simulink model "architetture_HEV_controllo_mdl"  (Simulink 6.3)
settings: Solver=ode45  StartTime=0.0  StopTime=8  RelTol=1e-3
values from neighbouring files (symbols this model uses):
  b_c = kb*J_c    (= 4.94590955184)    [architetture_epicicloidale.m]    (also in architetture_epicicloidale_cont.m; architetture_epicicloidale_HEV.m = 92.8974810391; architetture_epicicloidale_prova.m; architetture_HEV_controllo.m = 9.28974810391)
  b_p = kb*J_p    (= 8.12277148259)    [architetture_epicicloidale_HEV.m]    (also in architetture_HEV_controllo.m = 0.812277148259; architetture_HEV_startstop.m = 0.0731049433433; Confronto_CVT_EMR.m = 0; epicicloidale_confronto_statico_elastico.m)
  b_r = kb*J_r    (= 218.026030555)    [architetture_epicicloidale.m]    (also in architetture_epicicloidale_cont.m; architetture_epicicloidale_HEV.m; architetture_epicicloidale_prova.m; architetture_HEV_controllo.m = 21.8026030555)
  b_s = kb*J_s    (= 8.12277148259)    [architetture_epicicloidale.m]    (also in architetture_epicicloidale_cont.m; architetture_epicicloidale_HEV.m = 4.94590955184; architetture_epicicloidale_prova.m; architetture_HEV_controllo.m = 0.494590955184)
  bm = 0.8*N*metri*secondo/rad    (= 0.8)    [architetture_epicicloidale.m]    (also in architetture_epicicloidale_cont.m; architetture_epicicloidale_HEV.m; architetture_epicicloidale_prova.m; architetture_HEV_controllo.m)
  d_cr = d0    (= 10)    [architetture_epicicloidale_HEV.m]    (also in architetture_HEV_controllo.m = 1000; architetture_HEV_startstop.m = 90; epicicloidale_confronto_statico_elastico.m; epicicloidale_statico.m)
  d_sc = d0    (= 10)    [architetture_epicicloidale_HEV.m]    (also in architetture_HEV_controllo.m = 1000; architetture_HEV_startstop.m = 90; epicicloidale_confronto_statico_elastico.m; epicicloidale_statico.m)
  I_m = eye(m-1)    [architetture_epicicloidale.m]    (also in architetture_epicicloidale_cont.m; architetture_epicicloidale_HEV.m; architetture_epicicloidale_prova.m; architetture_HEV_controllo.m)
  Iw0 = 0*wI0    [architetture_epicicloidale.m]    (also in architetture_epicicloidale_cont.m = wI0; architetture_epicicloidale_HEV.m; architetture_epicicloidale_prova.m; architetture_HEV_controllo.m)
  J_c = 1.3*0.5*pi*rho_acc*hc*r_c^4    (= 0.0494590955184)    [architetture_epicicloidale.m]    (also in architetture_epicicloidale_cont.m; architetture_epicicloidale_HEV.m = 0.928974810391; architetture_epicicloidale_prova.m; architetture_HEV_controllo.m = 0.928974810391)
  J_p = Nr_sat*0.5*pi*rho_acc*(hs*r_p^4 + hc*r_p^4)    (= 0.0812277148259)    [architetture_epicicloidale_HEV.m]    (also in architetture_HEV_controllo.m; architetture_HEV_startstop.m; Confronto_CVT_EMR.m = 0; epicicloidale_confronto_statico_elastico.m)
  J_r = 0.5*pi*rho_acc*(hr*r_ri^4 + h_ring*(r_re^4-r_ri^4))    (= 2.18026030555)    [architetture_epicicloidale.m]    (also in architetture_epicicloidale_cont.m; architetture_epicicloidale_HEV.m; architetture_epicicloidale_prova.m; architetture_HEV_controllo.m)
  J_s = Nr_sat*0.5*pi*rho_acc*(hs*r_s^4 + hc*r_s^4)    (= 0.0812277148259)    [architetture_epicicloidale.m]    (also in architetture_epicicloidale_cont.m; architetture_epicicloidale_HEV.m = 0.0494590955184; architetture_epicicloidale_prova.m; architetture_HEV_controllo.m = 0.0494590955184)
  Jm = 1.6*kg*metri^2    (= 1.6)    [architetture_epicicloidale.m]    (also in architetture_epicicloidale_cont.m; architetture_epicicloidale_HEV.m = 1.64945909552; architetture_epicicloidale_prova.m; architetture_HEV_controllo.m = 0.529459095518)
  Jr = Jr([1:m-1],[1:m-1])    [architetture_epicicloidale.m]    (also in architetture_epicicloidale_cont.m; architetture_epicicloidale_HEV.m; architetture_epicicloidale_prova.m; architetture_HEV_controllo.m)
  K_cr = K0    (= 10000)    [architetture_epicicloidale_HEV.m]    (also in architetture_HEV_controllo.m = 100000; architetture_HEV_startstop.m = 10000000; epicicloidale_confronto_statico_elastico.m; epicicloidale_statico.m)
  K_sc = K0    (= 10000)    [architetture_epicicloidale_HEV.m]    (also in architetture_HEV_controllo.m = 100000; architetture_HEV_startstop.m = 10000000; epicicloidale_confronto_statico_elastico.m; epicicloidale_statico.m)
  Kf = diag(diag(MLb)'./fliplr(tau_m(1:m-1)))    [architetture_epicicloidale_cont.m]    (also in architetture_epicicloidale_HEV.m; architetture_epicicloidale_prova.m; architetture_HEV_controllo.m; architetture_HEV_startstop.m)
  Kr = Kr([1:m-1])    [architetture_epicicloidale.m]    (also in architetture_epicicloidale_cont.m; architetture_epicicloidale_HEV.m; architetture_epicicloidale_prova.m; architetture_HEV_controllo.m)
  Li = 0.1*Henry    (= 0.1)    [architetture_epicicloidale.m]    (also in architetture_epicicloidale_cont.m; architetture_epicicloidale_HEV.m; architetture_epicicloidale_prova.m; architetture_HEV_controllo.m)
  m = 5    [architetture_epicicloidale.m]    (also in architetture_epicicloidale_cont.m; architetture_epicicloidale_HEV.m; architetture_epicicloidale_prova.m; architetture_HEV_controllo.m)
  Mi = 0.08*Henry    (= 0.08)    [architetture_epicicloidale.m]    (also in architetture_epicicloidale_cont.m; architetture_epicicloidale_HEV.m; architetture_epicicloidale_prova.m; architetture_HEV_controllo.m)
  MKr = MKr([1:m-1],[1:m-1])    [architetture_epicicloidale.m]    (also in architetture_epicicloidale_cont.m; architetture_epicicloidale_HEV.m; architetture_epicicloidale_prova.m; architetture_HEV_controllo.m)
  MLb = MLb([1:m-1],[1:m-1])    [architetture_epicicloidale.m]    (also in architetture_epicicloidale_cont.m; architetture_epicicloidale_HEV.m; architetture_epicicloidale_prova.m; architetture_HEV_controllo.m)
  MR = MR([1:m-1],[1:m-1])    [architetture_epicicloidale.m]    (also in architetture_epicicloidale_cont.m; architetture_epicicloidale_HEV.m; architetture_epicicloidale_prova.m; architetture_HEV_controllo.m)
  Nar = 200    [architetture_epicicloidale.m]    (also in architetture_epicicloidale_cont.m; architetture_epicicloidale_HEV.m; architetture_epicicloidale_prova.m; architetture_HEV_controllo.m)
  Nc = 30    [architetture_epicicloidale.m]    (also in architetture_epicicloidale_cont.m; architetture_epicicloidale_HEV.m; architetture_epicicloidale_prova.m; architetture_HEV_controllo.m)
  Nr_sat = 4    [architetture_epicicloidale.m]    (also in architetture_epicicloidale_cont.m; architetture_epicicloidale_HEV.m; architetture_epicicloidale_prova.m; architetture_HEV_controllo.m)
  p = 1    [architetture_epicicloidale.m]    (also in architetture_epicicloidale_cont.m; architetture_epicicloidale_HEV.m; architetture_epicicloidale_prova.m; architetture_HEV_controllo.m)
  Phir = 0.02*Weber    (= 0.02)    [architetture_epicicloidale.m]    (also in architetture_epicicloidale_cont.m; architetture_epicicloidale_HEV.m; architetture_epicicloidale_prova.m; architetture_HEV_controllo.m)
  r_p = xds*Np/(2*pi)    (= 0.0732112738223)    [architetture_epicicloidale_HEV.m]    (also in architetture_HEV_controllo.m; architetture_HEV_startstop.m; Confronto_CVT_EMR.m = 0.025; epicicloidale_confronto_statico_elastico.m)
  r_r = xds*Nr/(2*pi)    (= 0.248281711223)    [architetture_epicicloidale_HEV.m]    (also in architetture_HEV_controllo.m; architetture_HEV_startstop.m; Confronto_CVT_EMR.m = 0.1; epicicloidale_confronto_statico_elastico.m)
  r_s = xds*Ns/(2*pi)    (= 0.0732112738223)    [architetture_epicicloidale.m]    (also in architetture_epicicloidale_cont.m; architetture_epicicloidale_HEV.m = 0.101859163579; architetture_epicicloidale_prova.m; architetture_HEV_controllo.m = 0.101859163579)
  Ri = 3*Ohm    (= 3)    [architetture_epicicloidale.m]    (also in architetture_epicicloidale_cont.m; architetture_epicicloidale_HEV.m; architetture_epicicloidale_prova.m; architetture_HEV_controllo.m = 0.1)
  Star = Si    [architetture_epicicloidale.m]    (also in architetture_epicicloidale_cont.m; architetture_epicicloidale_HEV.m; architetture_epicicloidale_prova.m; architetture_HEV_controllo.m)
  Tau_stop = 10000000    [architetture_HEV_controllo.m]
  Tc = 0.05*ms    (= 5e-05)    [architetture_epicicloidale.m]    (also in architetture_epicicloidale_cont.m; architetture_epicicloidale_HEV.m; architetture_epicicloidale_prova.m; architetture_HEV_controllo.m)
  Tc_0 = 0*N*metri    (= 0)    [architetture_epicicloidale_HEV.m]    (also in architetture_HEV_controllo.m; architetture_HEV_startstop.m; epicicloidale_confronto_statico_elastico.m; epicicloidale_statico.m)
  Thm0 = 0    [architetture_epicicloidale.m]    (also in architetture_epicicloidale_cont.m; architetture_epicicloidale_HEV.m; architetture_epicicloidale_prova.m; architetture_HEV_controllo.m)
  Tr_0 = 0*N*metri    (= 0)    [architetture_epicicloidale_HEV.m]    (also in architetture_HEV_controllo.m; architetture_HEV_startstop.m; epicicloidale_confronto_statico_elastico.m; epicicloidale_statico.m)
  Ts = Tfin/2000    (= 0.00025)    [architetture_epicicloidale.m]    (also in architetture_epicicloidale_cont.m = 0.001; architetture_epicicloidale_HEV.m = 0.0025; architetture_epicicloidale_prova.m = 0.001; architetture_HEV_controllo.m = 0.004)
  Ts_0 = 0*N*metri    (= 0)    [architetture_epicicloidale_HEV.m]    (also in architetture_HEV_controllo.m; architetture_HEV_startstop.m; epicicloidale_confronto_statico_elastico.m; epicicloidale_statico.m)
  tTb = tTb(:,[1:m-1])    [architetture_epicicloidale.m]    (also in architetture_epicicloidale_cont.m; architetture_epicicloidale_HEV.m; architetture_epicicloidale_prova.m; architetture_HEV_controllo.m)
  W_c = 100*rpm    (= 10.471975512)    [architetture_epicicloidale_HEV.m]    (also in architetture_HEV_controllo.m = 104.71975512; architetture_HEV_startstop.m = 0; PMSM_controllo_w.m; architetture_HEV_startstop_1.m = 0)
  Wm0 = 0*Wr_d    (= 0)    [architetture_epicicloidale.m]    (also in architetture_epicicloidale_cont.m = 62.5; architetture_epicicloidale_HEV.m; architetture_epicicloidale_prova.m; architetture_HEV_controllo.m)
undefined symbols (not defined in the file or in its folder): a_0, a_1, B_Pneumatico, DFKc_max, eps_sk, K_Pneumatico, Lambda_mu, Mass_Matrix, Massa_Corpo_Auto, Mu_lambda, Raggio_Ruota_Ant, Raggio_Ruota_Pos, T_omega, tau_a0
libraries: simulink x11, dspmtrx3 x4, Tire_Soil x2, planetary_gear_blocks x1, POG_Sincronous_Motors x1, dspstat3 x1

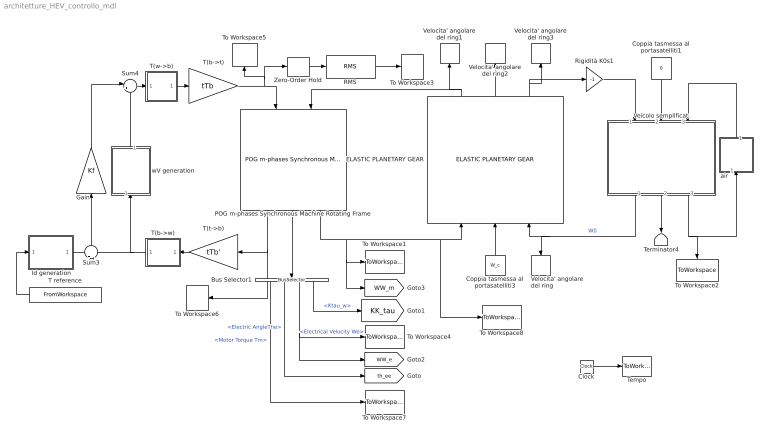
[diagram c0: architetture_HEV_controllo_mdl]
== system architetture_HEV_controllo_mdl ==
  " Id generation" : Subsystem
  Bus Selector1 : BusSelector  Orientation=down  OutputSignals=Motor Torque Tm,Electric AngleThe,Electrical Velocity We,Ktau_w
  Clock : Clock
  Coppia tasmessa al portasatelliti1 : Constant  Orientation=down  Value=0
  Coppia tasmessa al portasatelliti3 : Constant  Orientation=up  Value=W_c
  ELASTIC PLANETARY GEAR : planetary_gear_blocks/ELASTIC PLANETARY GEAR  Orientation=up  Par_solare=[J_s, b_s, r_s]  Par_satelliti=[J_p, J_c, b_p, b_c, r_p, Nr_sat]  Par_ring=[J_r, b_r, r_r]  Solare_Satelliti=[K_sc, d_sc]  Satelliti_Ring=[K_cr, d_cr]  Cond_in=[Ts_0, Tc_0, Tr_0]
  Gain : Gain  Orientation=up  Gain=Kf  Multiplication=Matrix(K*u) (u vector)
  POG m-phases Synchronous Machine Rotating Frame : POG_Sincronous_Motors/POG m-phases Synchronous Machine Rotating Frame  Orientation=down  Motor_Par=[m p]  Phase_Par=[Nc Star]  Electric_Par=[Ri Li Mi]  Mech_Par=[Jm bm]  Plux_Par=[Phir Nar]  Iniz_Cond=[Wm0; Thm0; Iw0]  TipoFlux=User defined  Tipo=Tipo  alfa=al  degree=6  TipoF=Tipo
  RMS : dspstat3/RMS  run=on  reset_popup=None
  Rigidità K0s1 : Gain  Gain=-1
  Sum3 : Sum  Orientation=up  Inputs=+|-
  Sum4 : Sum  Inputs=|++
  T reference : FromWorkspace  Orientation=left  VariableName=[T_in T_des]  SampleTime=0
  T(b->t) : Gain  Gain=tTb  Multiplication=Matrix(K*u) (u vector)
  T(b->w) : Subsystem  Orientation=left  AncestorBlock=|
      | POG_Electric_Bloks/POG m-phases
      | Synchronous Machine
      | Rotating Frame/T(b->w)
  T(t->b) : Gain  Orientation=left  Gain=tTb'  Multiplication=Matrix(K*u) (u vector)
  T(w->b) : Subsystem  AncestorBlock=|
      | POG_Electric_Bloks/POG m-phases
      | Synchronous Machine
      | Rotating Frame/T(w->b)
  Tempo : ToWorkspace  VariableName=t  SampleTime=Tc  SaveFormat=Array
  Terminator4 : Terminator
  To Workspace1 : ToWorkspace  VariableName=Wm  SampleTime=Tc  SaveFormat=Array
  To Workspace2 : ToWorkspace  VariableName=Vvehicle  SampleTime=Tc  SaveFormat=Array
  To Workspace3 : ToWorkspace  VariableName=Vt1  SampleTime=Tc  SaveFormat=Array
  To Workspace4 : ToWorkspace  VariableName=We  SampleTime=Tc  SaveFormat=Array
  To Workspace5 : ToWorkspace  VariableName=Vt  SampleTime=Tc  SaveFormat=Array
  To Workspace6 : ToWorkspace  VariableName=It  SampleTime=Tc  SaveFormat=Array
  To Workspace7 : ToWorkspace  VariableName=Tm  SampleTime=Tc  SaveFormat=Array
  To Workspace8 : ToWorkspace  VariableName=Ws  SampleTime=Tc  SaveFormat=Array
  Veicolo semplificat : Subsystem  Orientation=down
  Velocita' angolare del ring : ToWorkspace  VariableName=W_r  SampleTime=Tc  SaveFormat=Array
  Velocita' angolare del ring1 : ToWorkspace  VariableName=Tau_s  SampleTime=Tc  SaveFormat=Array
  Velocita' angolare del ring2 : ToWorkspace  VariableName=Tau_c  SampleTime=Tc  SaveFormat=Array
  Velocita' angolare del ring3 : ToWorkspace  VariableName=Tau_r  SampleTime=Tc  SaveFormat=Array
  Zero-Order Hold : ZeroOrderHold  SampleTime=Ts
  air : Subsystem  Orientation=up
  wV generation : Subsystem  Orientation=up
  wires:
  Clock/1 -> Tempo/1
  POG m-phases Synchronous Machine Rotating Frame/3 -> To Workspace1/1, [WW_m], ELASTIC PLANETARY GEAR/1, To Workspace8/1
  POG m-phases Synchronous Machine Rotating Frame/2 -> Bus Selector1/1
  Bus Selector1/3 -> To Workspace4/1, [WW_e]  "<Electrical Velocity We>"
  T(w->b)/1(It) -> T(b->t)/1
  T(b->t)/1 -> POG m-phases Synchronous Machine Rotating Frame/1, To Workspace5/1, Zero-Order Hold/1
  T(t->b)/1 -> T(b->w)/1(Vt)
  T(b->w)/1(Vw) -> wV generation/1(In1), Sum3/2
  POG m-phases Synchronous Machine Rotating Frame/1 -> T(t->b)/1, To Workspace6/1
  Bus Selector1/2 -> [th_ee]  "<Electric AngleThe>"
  Bus Selector1/1 -> To Workspace7/1  "<Motor Torque Tm>"
  Coppia tasmessa al portasatelliti1/1 -> Veicolo semplificat/2(Tau2)
  Rigidità K0s1/1 -> Veicolo semplificat/1(Tau1)
  " Id generation"/1(Out1) -> Sum3/1
  Sum3/1 -> Gain/1
  Sum4/1 -> T(w->b)/1(Iw)
  Gain/1 -> Sum4/1
  wV generation/1(Out1) -> Sum4/2
  Veicolo semplificat/3(V) -> To Workspace2/1, air/1(In1)
  Bus Selector1/4 -> [KK_tau]  "<Ktau_w>"
  air/1(Out1) -> Veicolo semplificat/3(Fres)
  Veicolo semplificat/2(W2) -> Terminator4/1
  ELASTIC PLANETARY GEAR/3 -> Velocita' angolare del ring3/1, Rigidità K0s1/1
  ELASTIC PLANETARY GEAR/1 -> Velocita' angolare del ring1/1, POG m-phases Synchronous Machine Rotating Frame/2
  ELASTIC PLANETARY GEAR/2 -> Velocita' angolare del ring2/1
  Coppia tasmessa al portasatelliti3/1 -> ELASTIC PLANETARY GEAR/2
  Veicolo semplificat/1(W1) -> Velocita' angolare del ring/1, ELASTIC PLANETARY GEAR/3  "W0"
  T reference/1 -> " Id generation"/1(In1)
  RMS/1 -> To Workspace3/1
  Zero-Order Hold/1 -> RMS/1

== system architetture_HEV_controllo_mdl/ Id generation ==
  In1 : Inport
  Divide : Product  Inputs=*/  OutScaling=2^-10
  Product : Product
  modulo : Subsystem
  versore : Subsystem
  Out1 : Outport
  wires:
  [KK_tau] -> modulo/1(In1), versore/1(In1)
  modulo/1(Out1) -> Divide/2
  Divide/1 -> Product/1
  versore/1(Out1) -> Product/2
  In1/1 -> Divide/1
  Product/1 -> Out1/1

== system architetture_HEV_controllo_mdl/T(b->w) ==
  Vt : Inport
  Product : Product  Multiplication=Matrix(*)
  Vw : Outport
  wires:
  Vt/1 -> Product/2
  Product/1 -> Vw/1
  [T_w_be] -> Product/1

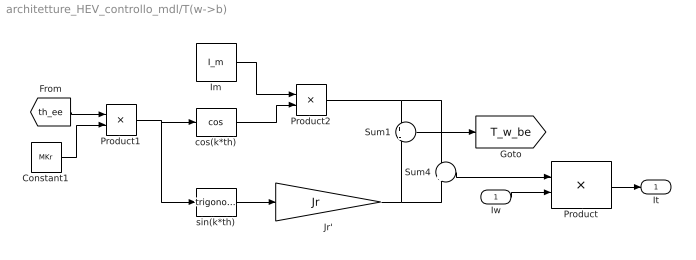
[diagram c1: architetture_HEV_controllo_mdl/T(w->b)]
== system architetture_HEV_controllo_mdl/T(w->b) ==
  Iw : Inport
  Constant1 : Constant  Value=MKr
  Im : Constant  Value=I_m  VectorParams1D=off
  Jr' : Gain  Gain=Jr  Multiplication=Matrix(K*u)
  Product : Product  Multiplication=Matrix(*)
  Product1 : Product
  Product2 : Product
  Sum1 : Sum  Inputs=+|-
  Sum4 : Sum  Inputs=+|+
  cos(k*th) : Trigonometry  Operator=cos
  sin(k*th) : Trigonometry
  It : Outport
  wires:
  Sum4/1 -> Product/1
  Product/1 -> It/1
  Iw/1 -> Product/2
  Jr'/1 -> Sum4/2, Sum1/2
  Product2/1 -> Sum4/1, Sum1/1
  Im/1 -> Product2/1
  cos(k*th)/1 -> Product2/2
  Product1/1 -> sin(k*th)/1, cos(k*th)/1
  Constant1/1 -> Product1/2
  [th_ee] -> Product1/1
  sin(k*th)/1 -> Jr'/1
  Sum1/1 -> [T_w_be]

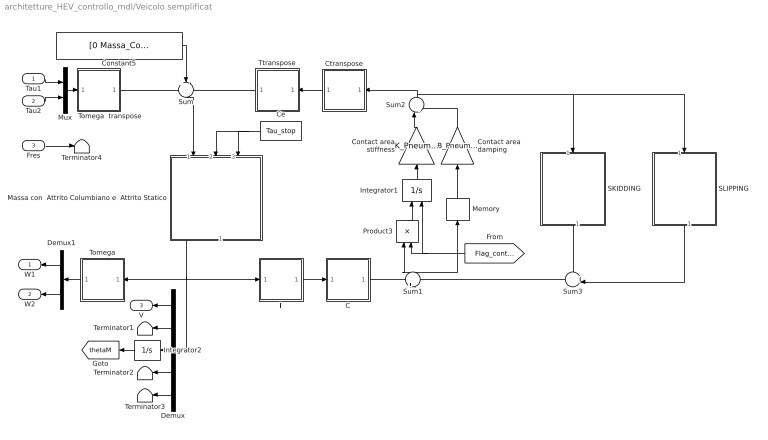
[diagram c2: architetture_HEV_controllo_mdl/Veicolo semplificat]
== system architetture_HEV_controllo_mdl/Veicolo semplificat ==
  Tau1 : Inport
  Tau2 : Inport  Port=2
  Fres : Inport  Port=3
  C : Subsystem
  Ce : Constant  Orientation=left  Value=Tau_stop
  Constant5 : Constant  Value=[0 Massa_Corpo_Auto*9.81 0 0 0]
  Contact area damping : Gain  Orientation=up  Gain=B_Pneumatico  Multiplication=Matrix(K*u) (u vector)
  Contact area stiffness : Gain  Orientation=up  Gain=K_Pneumatico  Multiplication=Matrix(K*u) (u vector)
  Ctranspose : Subsystem  Orientation=left
  Demux : Demux  Orientation=left  Outputs=5
  Demux1 : Demux  Orientation=left  Outputs=2
  Integrator1 : Integrator  Orientation=up  ExternalReset=falling  InitialCondition=[0 0 0 0 0 0]
  Integrator2 : Integrator  Orientation=left
  Massa con  Attrito Columbiano e  Attrito Statico : Subsystem  Orientation=down  mask(Massa con attrito columbiano){m=Mass_Matrix, b=0, Vx0=0}
      mask prompts: m "Massa  dell' elemento che trasla  [m] -> [kg]"; b "Coefficiente  di attrito lineare [b] -> [N*s/m]"; Vx0 "Velocità iniziale della massa [Vx0] -> [m*s]"
      mask help: F = Forza totale agente sulla massa Nc = Ampiezza dell'attrito columbiano Ns = Ampiezza dell'attrito di primo distacco (Ns>Nc) m = Massa dell' elemento che trasla [kg] b = Coefficiente di attrito lineare [N*s/m] Vx0 = Velocità iniziale della massa [m*s]
  Memory : Memory  Orientation=up
  Mux : Mux  Inputs=2
  Product3 : Product  Orientation=up  Inputs=**
  SKIDDING : Subsystem  Orientation=down  AncestorBlock=Tire_Soil/Tire-soil contact ENERGETIC/Contatto elastico/SKIDDING
  SLIPPING : Subsystem  Orientation=down  AncestorBlock=Tire_Soil/Tire-soil contact ENERGETIC/Contatto elastico/SLIPPING
  Sum : Sum  Orientation=down  Inputs=+--
  Sum1 : Sum  Orientation=up  Inputs=+-
  Sum2 : Sum  Orientation=up  Inputs=|++
  Sum3 : Sum  Orientation=left  Inputs=++|
  T : Subsystem
  Terminator{1..4} (4 alike) : Terminator
  Tomega : Subsystem  Orientation=left
  Tomega  transpose : Subsystem
  Ttranspose : Subsystem  Orientation=left
  W1 : Outport  Orientation=left
  W2 : Outport  Orientation=left  Port=2
  V : Outport  Orientation=left  Port=3
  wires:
  Demux/5 -> Terminator3/1
  Demux/4 -> Terminator2/1
  Demux/2 -> Terminator1/1
  Demux/1 -> V/1
  Tomega/1(Vt) -> Demux1/1
  Tau2/1 -> Mux/2
  Tau1/1 -> Mux/1
  Mux/1 -> Tomega  transpose/1(T)
  Tomega  transpose/1(Tt) -> Sum/1
  Constant5/1 -> Sum/2
  Sum3/1 -> Sum1/2
  SKIDDING/1(Vcsk) -> Sum3/1
  SLIPPING/1(Vcsl) -> Sum3/2
  Memory/1 -> Contact area damping/1
  Integrator1/1 -> Contact area stiffness/1
  Product3/1 -> Integrator1/1
  [Flag_contatto] -> Integrator1/2, Product3/2
  C/1(Xcdot) -> Sum1/1
  Ctranspose/1(F) -> Ttranspose/1(F)
  T/1(Xdot) -> C/1(Xdot)
  Integrator2/1 -> [thetaM]
  Demux/3 -> Integrator2/1
  Contact area stiffness/1 -> Sum2/1
  Contact area damping/1 -> Sum2/2
  Sum1/1 -> Memory/1, Product3/1
  Sum2/1 -> Ctranspose/1(Fc), SLIPPING/1(Fxyz), SKIDDING/1(Fxyz)
  Ttranspose/1(Ft) -> Sum/3
  Massa con  Attrito Columbiano e  Attrito Statico/1(Vx) -> Tomega/1(V), Demux/1, T/1(V)
  Sum/1 -> Massa con  Attrito Columbiano e  Attrito Statico/1(F)
  Demux1/1 -> W1/1
  Demux1/2 -> W2/1
  Fres/1 -> Terminator4/1
  Ce/1 -> Massa con  Attrito Columbiano e  Attrito Statico/2(Nc), Massa con  Attrito Columbiano e  Attrito Statico/3(Ns)

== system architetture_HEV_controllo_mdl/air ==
  In1 : Inport  Orientation=up
  air : Fcn  Orientation=up  Expr=10*u^2
  Out1 : Outport  Orientation=up
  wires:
  In1/1 -> air/1
  air/1 -> Out1/1

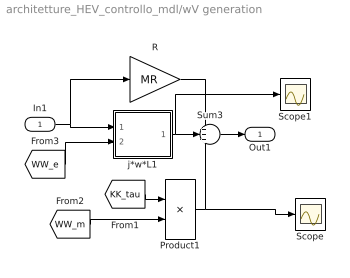
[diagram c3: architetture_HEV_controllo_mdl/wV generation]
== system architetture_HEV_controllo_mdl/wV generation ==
  In1 : Inport
  Product1 : Product  Multiplication=Matrix(*)
  R : Gain  Gain=MR  Multiplication=Matrix(K*u) (u vector)
  Scope : Scope
  Scope1 : Scope
  Sum3 : Sum  Inputs=+++
  j*w*L1 : Subsystem  AncestorBlock=|
      | POG_Electric_Bloks/POG m-phases
      | Synchronous Machine
      | Rotating Frame/j*w*L
  Out1 : Outport
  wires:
  [KK_tau] -> Product1/1
  [WW_m] -> Product1/2
  R/1 -> Sum3/1
  j*w*L1/1(Out1) -> Sum3/2, Scope1/1
  Product1/1 -> Sum3/3, Scope/1
  In1/1 -> j*w*L1/1(In1), R/1
  Sum3/1 -> Out1/1
  [WW_e] -> j*w*L1/2(In2)

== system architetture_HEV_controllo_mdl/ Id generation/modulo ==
  In1 : Inport
  Dot Product : simulink/Math Operations/Dot Product  InputSameDT=on  OutDataType=sfix(16)  OutScaling=2^-10  DoSatur=off
  Math Function : Math  Operator=sqrt
  Out1 : Outport
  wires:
  In1/1 -> Dot Product/1, Dot Product/2
  Dot Product/1 -> Math Function/1
  Math Function/1 -> Out1/1

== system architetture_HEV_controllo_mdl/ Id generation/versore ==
  In1 : Inport
  Constant : Constant  Value=0.0001
  Divide : Product  Inputs=*/  OutScaling=2^-10
  Norma  del vettore : Subsystem
  Sum1 : Sum  Inputs=|++
  Out1 : Outport
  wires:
  Divide/1 -> Out1/1  "versore"
  Constant/1 -> Sum1/2
  Sum1/1 -> Divide/2
  Norma  del vettore/1(Out1) -> Sum1/1
  In1/1 -> Norma  del vettore/1(In1), Divide/1

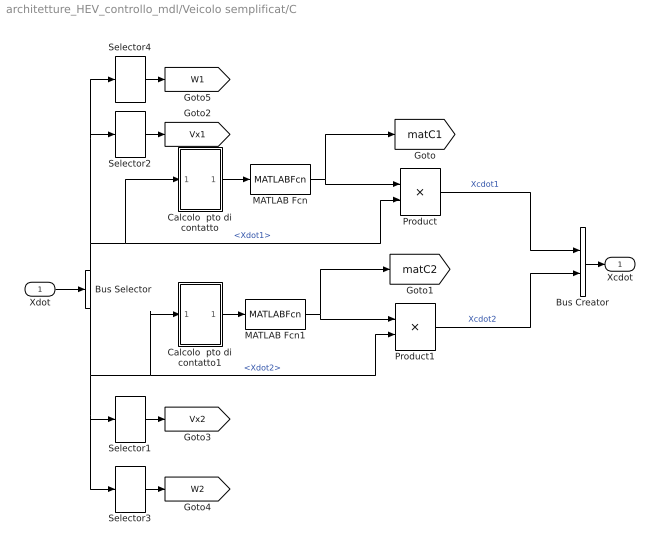
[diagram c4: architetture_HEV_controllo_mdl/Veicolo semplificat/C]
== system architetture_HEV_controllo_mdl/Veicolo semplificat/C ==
  Xdot : Inport
  Bus Creator : BusCreator  Inputs=2
  Bus Selector : BusSelector  OutputSignals=Xdot1,Xdot2
  Calcolo  pto di contatto : Subsystem
  Calcolo  pto di contatto1 : Subsystem
  MATLAB Fcn : MATLABFcn  MATLABFcn=matrice_c  Output1D=off
  MATLAB Fcn1 : MATLABFcn  MATLABFcn=matrice_c  Output1D=off
  Product : Product  Inputs=**  Multiplication=Matrix(*)
  Product1 : Product  Inputs=**  Multiplication=Matrix(*)
  Selector1 : Selector  InputPortWidth=3
  Selector2 : Selector  InputPortWidth=3
  Selector3 : Selector  Elements=3  InputPortWidth=3
  Selector4 : Selector  Elements=3  InputPortWidth=3
  Xcdot : Outport
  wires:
  Selector3/1 -> [W2]
  Selector4/1 -> [W1]
  Selector1/1 -> [Vx2]
  Selector2/1 -> [Vx1]
  Bus Creator/1 -> Xcdot/1
  Bus Selector/1 -> Selector4/1, Selector2/1, Product/2, Calcolo  pto di contatto/1(In1)  "<Xdot1>"
  Xdot/1 -> Bus Selector/1
  Calcolo  pto di contatto1/1(Out1) -> MATLAB Fcn1/1
  MATLAB Fcn1/1 -> [matC2], Product1/1
  Bus Selector/2 -> Selector3/1, Selector1/1, Calcolo  pto di contatto1/1(In1), Product1/2  "<Xdot2>"
  Product1/1 -> Bus Creator/2  "Xcdot2"
  Calcolo  pto di contatto/1(Out1) -> MATLAB Fcn/1
  MATLAB Fcn/1 -> [matC1], Product/1
  Product/1 -> Bus Creator/1  "Xcdot1"

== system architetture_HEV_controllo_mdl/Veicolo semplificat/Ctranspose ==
  Fc : Inport
  Mux : Mux  Inputs=2
  Product : Product  Inputs=**  Multiplication=Matrix(*)
  Product1 : Product  Inputs=**  Multiplication=Matrix(*)
  Selector : Selector  Elements=[1 2 3]  InputPortWidth=6
  Selector1 : Selector  Elements=[4 5 6]  InputPortWidth=6
  Transpose : dspmtrx3/Transpose  Hermitian=off  overflowFlag=on
  Transpose1 : dspmtrx3/Transpose  Hermitian=off  overflowFlag=on
  F : Outport
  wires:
  Selector1/1 -> Product1/2
  Selector/1 -> Product/2
  Fc/1 -> Selector1/1, Selector/1
  Mux/1 -> F/1
  Product1/1 -> Mux/2
  Product/1 -> Mux/1
  [matC2] -> Transpose1/1
  Transpose1/1 -> Product1/1
  [matC1] -> Transpose/1
  Transpose/1 -> Product/1

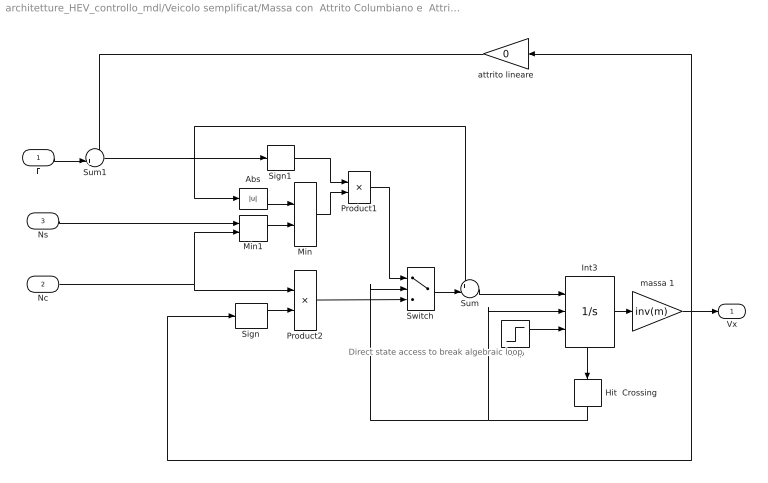
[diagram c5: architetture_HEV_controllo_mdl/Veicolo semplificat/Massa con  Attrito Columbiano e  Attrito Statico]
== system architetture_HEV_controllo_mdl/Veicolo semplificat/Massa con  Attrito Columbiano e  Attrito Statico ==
  note: Direct state access to break algebraic loop
  F : Inport
  Nc : Inport  Port=2
  Ns : Inport  Port=3
  Abs : Abs
  Hit  Crossing : HitCross  Orientation=down
  Int3 : Integrator  ExternalReset=rising  InitialConditionSource=external  InitialCondition=Vx0  ShowStatePort=on
  Min : MinMax  Inputs=2
  Min1 : MinMax  Function=max  Inputs=2
  Product1 : Product
  Product2 : Product
  Sign : Signum
  Sign1 : Signum
  Step : Step  Time=0.0000001  After=0  SampleTime=0  ZeroCross=off
  Sum : Sum  Inputs=+-|
  Sum1 : Sum  Inputs=-+|
  Switch : Switch  Threshold=0.5
  attrito lineare : Gain  Orientation=left  Gain=0
  massa 1 : Gain  Gain=inv(m)  Multiplication=Matrix(K*u) (u vector)
  Vx : Outport  InitialOutput=0
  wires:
  Product1/1 -> Switch/1
  Switch/1 -> Sum/2
  Hit  Crossing/1 -> Switch/2, Int3/2
  Sum1/1 -> Abs/1, Sign1/1, Sum/1
  Sum/1 -> Int3/1
  Int3/State -> Hit  Crossing/1
  Int3/1 -> massa 1/1
  Product2/1 -> Switch/3
  Nc/1 -> Product2/1, Min1/2
  Sign/1 -> Product2/2
  Sign1/1 -> Product1/1
  Min/1 -> Product1/2
  Abs/1 -> Min/1
  Min1/1 -> Min/2
  Ns/1 -> Min1/1
  attrito lineare/1 -> Sum1/1
  F/1 -> Sum1/2
  Step/1 -> Int3/3
  massa 1/1 -> Vx/1, attrito lineare/1, Sign/1

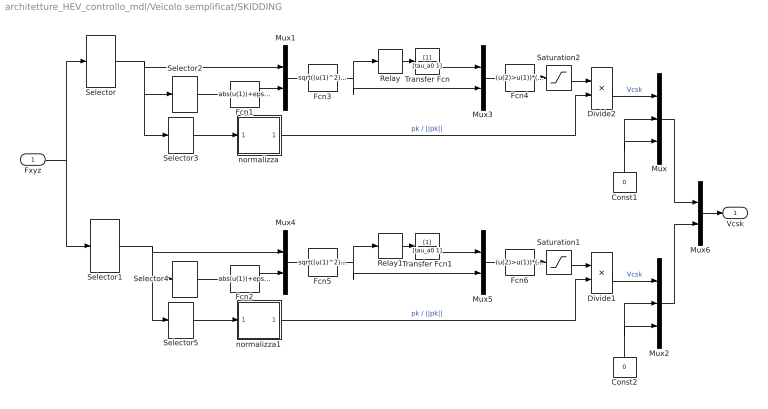
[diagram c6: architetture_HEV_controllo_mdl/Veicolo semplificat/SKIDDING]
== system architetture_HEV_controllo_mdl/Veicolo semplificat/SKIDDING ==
  Fxyz : Inport
  Const1 : Constant  Orientation=up  Value=0
  Const2 : Constant  Orientation=up  Value=0
  Divide1 : Product  Inputs=**  OutScaling=2^-10
  Divide2 : Product  Inputs=**  OutScaling=2^-10
  Fcn1 : Fcn  Expr=abs(u(1))+eps_sk
  Fcn2 : Fcn  Expr=abs(u(1))+eps_sk
  Fcn3 : Fcn  Expr=sqrt((u(1)^2))/u(4)
  Fcn4 : Fcn  Expr=(u(2)>u(1))*(u(2)-u(1))^2*Kc
  Fcn5 : Fcn  Expr=sqrt((u(1)^2))/u(4)
  Fcn6 : Fcn  Expr=(u(2)>u(1))*(u(2)-u(1))^2*Kc
  Mux : Mux  Inputs=3
  Mux{1,3..6} (5 alike) : Mux  Inputs=2
  Mux2 : Mux  Inputs=3
  Relay : Relay  OnSwitchValue=a_0  OffSwitchValue=a_1  OnOutputValue=a_1  OffOutputValue=a_0
  Relay1 : Relay  OnSwitchValue=a_0  OffSwitchValue=a_1  OnOutputValue=a_1  OffOutputValue=a_0
  Saturation1 : Saturate  UpperLimit=DFKc_max  LowerLimit=0
  Saturation2 : Saturate  UpperLimit=DFKc_max  LowerLimit=0
  Selector : Selector  Elements=[1 2 3]  InputPortWidth=6
  Selector1 : Selector  Elements=[4 5 6]  InputPortWidth=6
  Selector2 : Selector  Elements=[2]  InputPortWidth=3
  Selector3 : Selector  InputPortWidth=3
  Selector4 : Selector  Elements=[2]  InputPortWidth=3
  Selector5 : Selector  InputPortWidth=3
  Transfer Fcn : TransferFcn  Denominator=[tau_a0 1]
  Transfer Fcn1 : TransferFcn  Denominator=[tau_a0 1]
  normalizza : Subsystem
  normalizza1 : Subsystem
  Vcsk : Outport
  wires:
  Mux6/1 -> Vcsk/1
  Mux2/1 -> Mux6/2
  Mux/1 -> Mux6/1
  Const2/1 -> Mux2/3, Mux2/2
  Selector1/1 -> Mux4/1, Selector5/1, Selector4/1
  Divide1/1 -> Mux2/1  "Vcsk"
  Selector4/1 -> Fcn2/1
  Selector5/1 -> normalizza1/1(In1)
  normalizza1/1(Out1) -> Divide1/2  "pk / ||pk||"
  Saturation1/1 -> Divide1/1
  Fcn6/1 -> Saturation1/1
  Fcn5/1 -> Relay1/1, Mux5/2
  Mux4/1 -> Fcn5/1
  Fcn2/1 -> Mux4/2
  Mux5/1 -> Fcn6/1
  Relay1/1 -> Transfer Fcn1/1
  Transfer Fcn1/1 -> Mux5/1
  Const1/1 -> Mux/3, Mux/2
  Selector/1 -> Mux1/1, Selector3/1, Selector2/1
  Divide2/1 -> Mux/1  "Vcsk"
  Fxyz/1 -> Selector1/1, Selector/1
  Selector2/1 -> Fcn1/1
  Selector3/1 -> normalizza/1(In1)
  normalizza/1(Out1) -> Divide2/2  "pk / ||pk||"
  Saturation2/1 -> Divide2/1
  Fcn4/1 -> Saturation2/1
  Fcn3/1 -> Relay/1, Mux3/2
  Mux1/1 -> Fcn3/1
  Fcn1/1 -> Mux1/2
  Mux3/1 -> Fcn4/1
  Relay/1 -> Transfer Fcn/1
  Transfer Fcn/1 -> Mux3/1

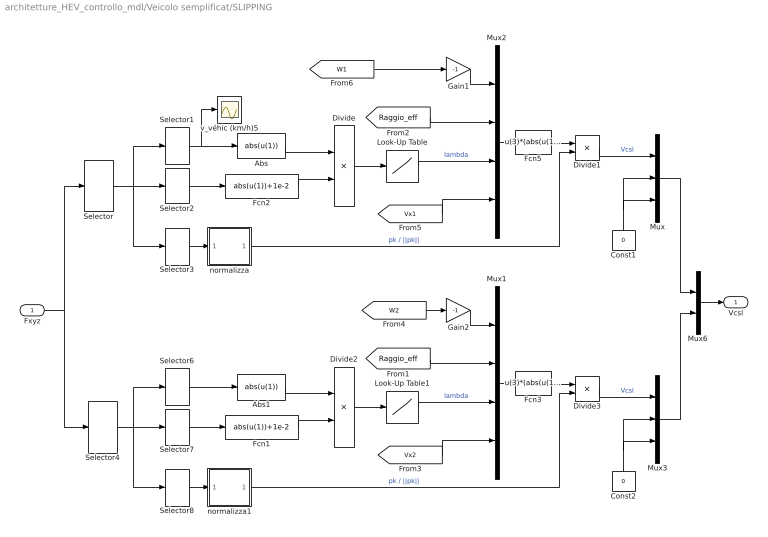
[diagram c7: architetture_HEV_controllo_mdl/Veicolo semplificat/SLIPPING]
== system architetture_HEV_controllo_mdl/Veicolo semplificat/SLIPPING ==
  Fxyz : Inport
  Abs : Fcn  Expr=abs(u(1))
  Abs1 : Fcn  Expr=abs(u(1))
  Const1 : Constant  Orientation=up  Value=0
  Const2 : Constant  Orientation=up  Value=0
  Divide : Product  Inputs=*/  OutScaling=2^-10
  Divide1 : Product  Inputs=**  OutScaling=2^-10
  Divide2 : Product  Inputs=*/  OutScaling=2^-10
  Divide3 : Product  Inputs=**  OutScaling=2^-10
  Fcn1 : Fcn  Expr=abs(u(1))+1e-2
  Fcn2 : Fcn  Expr=abs(u(1))+1e-2
  Fcn3 : Fcn  Expr=u(3)*(abs(u(1)*u(2))*(abs(u(1)*u(2))<=abs(u(4)))+abs(u(4))*(abs(u(1)*u(2))>abs(u(4))))
  Fcn5 : Fcn  Expr=u(3)*(abs(u(1)*u(2))*(abs(u(1)*u(2))<=abs(u(4)))+abs(u(4))*(abs(u(1)*u(2))>abs(u(4))))
  Gain1 : Gain  Gain=-1
  Gain2 : Gain  Gain=-1
  Look-Up Table : Lookup  InputValues=Mu_lambda  OutputValues=Lambda_mu
  Look-Up Table1 : Lookup  InputValues=Mu_lambda  OutputValues=Lambda_mu
  Mux : Mux  Inputs=3
  Mux1 : Mux
  Mux2 : Mux
  Mux3 : Mux  Inputs=3
  Mux6 : Mux  Inputs=2
  Selector : Selector  Elements=[1 2 3]  InputPortWidth=6
  Selector{1,3,6,8} (4 alike) : Selector  InputPortWidth=3
  Selector2 : Selector  Elements=[2]  InputPortWidth=3
  Selector4 : Selector  Elements=[4 5 6]  InputPortWidth=6
  Selector7 : Selector  Elements=[2]  InputPortWidth=3
  normalizza : Subsystem
  normalizza1 : Subsystem
  v_véhic (km/h)5 : Scope
  Vcsl : Outport
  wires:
  [W2] -> Gain2/1
  [W1] -> Gain1/1
  Mux6/1 -> Vcsl/1
  Mux3/1 -> Mux6/2
  Mux/1 -> Mux6/1
  Const2/1 -> Mux3/3, Mux3/2
  Divide3/1 -> Mux3/1  "Vcsl"
  Const1/1 -> Mux/2, Mux/3
  Divide1/1 -> Mux/1  "Vcsl"
  normalizza1/1(Out1) -> Divide3/2  "pk / ||pk||"
  Selector4/1 -> Selector6/1, Selector8/1, Selector7/1
  Selector7/1 -> Fcn1/1
  Selector8/1 -> normalizza1/1(In1)
  Fcn1/1 -> Divide2/2
  Abs1/1 -> Divide2/1
  Selector6/1 -> Abs1/1
  Look-Up Table1/1 -> Mux1/3  "lambda"
  Divide2/1 -> Look-Up Table1/1
  [Raggio_eff] -> Mux1/2
  Gain2/1 -> Mux1/1
  [Vx2] -> Mux1/4
  Mux1/1 -> Fcn3/1
  Fcn3/1 -> Divide3/1
  Fxyz/1 -> Selector4/1, Selector/1
  normalizza/1(Out1) -> Divide1/2  "pk / ||pk||"
  Selector/1 -> Selector1/1, Selector3/1, Selector2/1
  Selector2/1 -> Fcn2/1
  Selector3/1 -> normalizza/1(In1)
  Fcn2/1 -> Divide/2
  Abs/1 -> Divide/1
  Selector1/1 -> v_véhic (km/h)5/1, Abs/1
  Look-Up Table/1 -> Mux2/3  "lambda"
  Divide/1 -> Look-Up Table/1
  [Raggio_eff] -> Mux2/2
  Gain1/1 -> Mux2/1
  [Vx1] -> Mux2/4
  Mux2/1 -> Fcn5/1
  Fcn5/1 -> Divide1/1

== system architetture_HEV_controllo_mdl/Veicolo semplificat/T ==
  V : Inport
  Bus Creator : BusCreator  Inputs=2
  MATLAB Fcn : MATLABFcn  MATLABFcn=matrice_T  Output1D=off
  Product : Product  Inputs=**  Multiplication=Matrix(*)
  Selector : Selector  Elements=[1 2 3]  InputPortWidth=6
  Selector1 : Selector  Elements=[4 5 6]  InputPortWidth=6
  Xdot : Outport
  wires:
  Bus Creator/1 -> Xdot/1
  Selector/1 -> Bus Creator/1  "Xdot1"
  Selector1/1 -> Bus Creator/2  "Xdot2"
  Product/1 -> Selector1/1, Selector/1
  MATLAB Fcn/1 -> [matT], Product/1
  V/1 -> Product/2
  [thetaM] -> MATLAB Fcn/1

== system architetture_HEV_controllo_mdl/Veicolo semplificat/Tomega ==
  V : Inport
  Constant5 : Constant  Value=T_omega
  Product : Product  Inputs=**  Multiplication=Matrix(*)
  Vt : Outport
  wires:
  Product/1 -> Vt/1
  V/1 -> Product/2
  Constant5/1 -> Product/1

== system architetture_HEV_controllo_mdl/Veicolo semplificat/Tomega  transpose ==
  T : Inport
  Constant5 : Constant  Value=T_omega
  Product : Product  Inputs=**  Multiplication=Matrix(*)
  Transpose : dspmtrx3/Transpose  Hermitian=off  overflowFlag=on
  Tt : Outport
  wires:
  Transpose/1 -> Product/1
  Constant5/1 -> Transpose/1
  T/1 -> Product/2
  Product/1 -> Tt/1

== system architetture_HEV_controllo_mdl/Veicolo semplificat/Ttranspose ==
  F : Inport
  Product : Product  Inputs=**  Multiplication=Matrix(*)
  Transpose : dspmtrx3/Transpose  Hermitian=off  overflowFlag=on
  Ft : Outport
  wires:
  Transpose/1 -> Product/1
  [matT] -> Transpose/1
  F/1 -> Product/2
  Product/1 -> Ft/1

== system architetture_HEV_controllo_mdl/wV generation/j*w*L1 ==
  In1 : Inport
  In2 : Inport  Port=2
  Gain1 : Gain  Gain=Kr  Multiplication=Matrix(K*u) (u vector)
  Gain2 : Gain  Gain=Jr  Multiplication=Matrix(K*u) (u vector)
  Gain4 : Gain  Gain=MLb  Multiplication=Matrix(K*u) (u vector)
  Product : Product
  Out1 : Outport
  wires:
  In1/1 -> Gain4/1
  In2/1 -> Gain1/1
  Gain1/1 -> Product/1
  Gain4/1 -> Product/2
  Product/1 -> Gain2/1
  Gain2/1 -> Out1/1

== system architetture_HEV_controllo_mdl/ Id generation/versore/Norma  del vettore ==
  In1 : Inport
  Dot Product : simulink/Math Operations/Dot Product  InputSameDT=on  OutDataType=sfix(16)  OutScaling=2^-10  DoSatur=off
  Math Function : Math  Operator=sqrt
  Out1 : Outport
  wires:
  Math Function/1 -> Out1/1
  Dot Product/1 -> Math Function/1
  In1/1 -> Dot Product/2, Dot Product/1

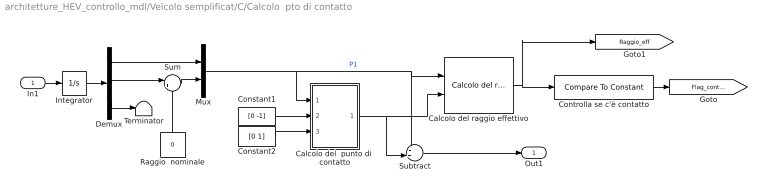
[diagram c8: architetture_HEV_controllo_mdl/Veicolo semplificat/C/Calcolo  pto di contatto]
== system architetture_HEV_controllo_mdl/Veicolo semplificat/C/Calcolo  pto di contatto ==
  In1 : Inport
  Calcolo del  punto di  contatto : Subsystem  AncestorBlock=|
      | Tire_Soil/Tire-soil contact
      | ENERGETIC/Calcolo versori
      | e punto di contatto C/Subsystem2/Calcolo del 
      | punto di 
      | contatto
  Calcolo del raggio effettivo : Tire_Soil/Tire-soil contact ENERGETIC/Calcolo versori e punto di contatto C/Subsystem2/Calcolo del raggio effettivo
  Constant1 : Constant  Value=[0 -1]
  Constant2 : Constant  Value=[0 1]
  Controlla se c'è contatto : simulink/Logic and Bit Operations/Compare To Constant  relop=<  const=Raggio_Ruota_Ant  LogicOutDataTypeMode=boolean  ZeroCross=off
  Demux : Demux  Outputs=3
  Integrator : Integrator  InitialCondition=[0 Raggio_Ruota_Pos 0]
  Mux : Mux  Inputs=2
  Raggio  nominale : Constant  Orientation=up  Value=0
  Subtract : Sum  Inputs=-+|  OutScaling=2^-10
  Sum : Sum  Inputs=|++
  Terminator : Terminator
  Out1 : Outport
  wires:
  Controlla se c'è contatto/1 -> [Flag_contatto]
  In1/1 -> Integrator/1
  Calcolo del raggio effettivo/1 -> [Raggio_eff], Controlla se c'è contatto/1
  Mux/1 -> Calcolo del  punto di  contatto/1(P1), Calcolo del raggio effettivo/1, Subtract/1  "P1"
  Constant1/1 -> Calcolo del  punto di  contatto/2(r)
  Calcolo del  punto di  contatto/1(Pc) -> Subtract/2, Calcolo del raggio effettivo/2
  Subtract/1 -> Out1/1
  Constant2/1 -> Calcolo del  punto di  contatto/3(n)
  Integrator/1 -> Demux/1
  Sum/1 -> Mux/2
  Demux/1 -> Mux/1
  Raggio  nominale/1 -> Sum/2
  Demux/2 -> Sum/1
  Demux/3 -> Terminator/1

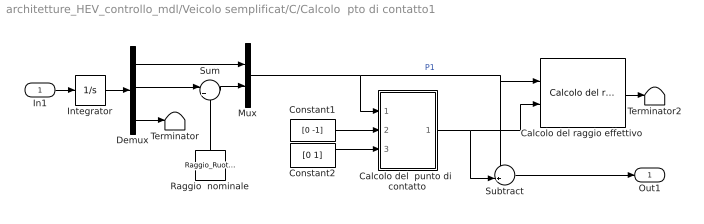
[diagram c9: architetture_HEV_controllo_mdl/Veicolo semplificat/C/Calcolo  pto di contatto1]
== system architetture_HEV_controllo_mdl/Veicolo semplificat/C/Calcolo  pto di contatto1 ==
  In1 : Inport
  Calcolo del  punto di  contatto : Subsystem  AncestorBlock=|
      | Tire_Soil/Tire-soil contact
      | ENERGETIC/Calcolo versori
      | e punto di contatto C/Subsystem2/Calcolo del 
      | punto di 
      | contatto
  Calcolo del raggio effettivo : Tire_Soil/Tire-soil contact ENERGETIC/Calcolo versori e punto di contatto C/Subsystem2/Calcolo del raggio effettivo
  Constant1 : Constant  Value=[0 -1]
  Constant2 : Constant  Value=[0 1]
  Demux : Demux  Outputs=3
  Integrator : Integrator
  Mux : Mux  Inputs=2
  Raggio  nominale : Constant  Orientation=up  Value=Raggio_Ruota_Pos
  Subtract : Sum  Inputs=-+|  OutScaling=2^-10
  Sum : Sum  Inputs=|++
  Terminator : Terminator
  Terminator2 : Terminator
  Out1 : Outport
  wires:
  In1/1 -> Integrator/1
  Calcolo del raggio effettivo/1 -> Terminator2/1
  Mux/1 -> Calcolo del  punto di  contatto/1(P1), Calcolo del raggio effettivo/1, Subtract/1  "P1"
  Constant1/1 -> Calcolo del  punto di  contatto/2(r)
  Calcolo del  punto di  contatto/1(Pc) -> Calcolo del raggio effettivo/2, Subtract/2
  Subtract/1 -> Out1/1
  Constant2/1 -> Calcolo del  punto di  contatto/3(n)
  Integrator/1 -> Demux/1
  Sum/1 -> Mux/2
  Demux/1 -> Mux/1
  Raggio  nominale/1 -> Sum/2
  Demux/2 -> Sum/1
  Demux/3 -> Terminator/1

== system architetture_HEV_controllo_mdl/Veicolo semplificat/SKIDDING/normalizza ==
  In1 : Inport
  Constant : Constant  Value=eps
  Divide : Product  Inputs=*/  OutScaling=2^-10
  Norma  del vettore : Subsystem
  Sum1 : Sum  Inputs=|++
  Out1 : Outport
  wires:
  In1/1 -> Divide/1, Norma  del vettore/1(In1)
  Norma  del vettore/1(Out1) -> Sum1/1
  Sum1/1 -> Divide/2
  Constant/1 -> Sum1/2
  Divide/1 -> Out1/1  "versore"

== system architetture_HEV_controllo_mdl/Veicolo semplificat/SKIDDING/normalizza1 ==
  In1 : Inport
  Constant : Constant  Value=eps
  Divide : Product  Inputs=*/  OutScaling=2^-10
  Norma  del vettore : Subsystem
  Sum1 : Sum  Inputs=|++
  Out1 : Outport
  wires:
  In1/1 -> Divide/1, Norma  del vettore/1(In1)
  Norma  del vettore/1(Out1) -> Sum1/1
  Sum1/1 -> Divide/2
  Constant/1 -> Sum1/2
  Divide/1 -> Out1/1  "versore"

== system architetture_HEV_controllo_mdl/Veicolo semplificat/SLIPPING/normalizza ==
  In1 : Inport
  Constant : Constant  Value=eps
  Divide : Product  Inputs=*/  OutScaling=2^-10
  Norma  del vettore : Subsystem
  Sum1 : Sum  Inputs=|++
  Out1 : Outport
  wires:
  In1/1 -> Divide/1, Norma  del vettore/1(In1)
  Norma  del vettore/1(Out1) -> Sum1/1
  Sum1/1 -> Divide/2
  Constant/1 -> Sum1/2
  Divide/1 -> Out1/1  "versore"

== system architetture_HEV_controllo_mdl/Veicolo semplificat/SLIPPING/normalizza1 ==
  In1 : Inport
  Constant : Constant  Value=eps
  Divide : Product  Inputs=*/  OutScaling=2^-10
  Norma  del vettore : Subsystem
  Sum1 : Sum  Inputs=|++
  Out1 : Outport
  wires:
  In1/1 -> Divide/1, Norma  del vettore/1(In1)
  Norma  del vettore/1(Out1) -> Sum1/1
  Sum1/1 -> Divide/2
  Constant/1 -> Sum1/2
  Divide/1 -> Out1/1  "versore"

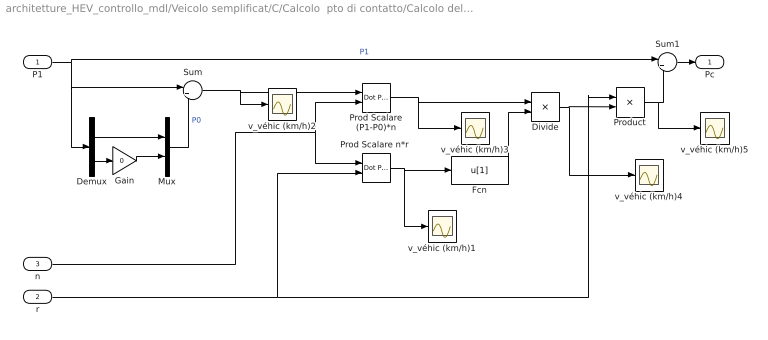
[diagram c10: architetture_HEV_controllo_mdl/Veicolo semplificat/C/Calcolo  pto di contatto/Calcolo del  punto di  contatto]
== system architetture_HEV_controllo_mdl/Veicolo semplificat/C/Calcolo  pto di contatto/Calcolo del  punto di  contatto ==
  P1 : Inport
  r : Inport  Port=2
  n : Inport  Port=3
  Demux : Demux  Outputs=2
  Divide : Product  Inputs=*/  OutScaling=2^-10
  Fcn : Fcn  Expr=u[1]
  Gain : Gain  Gain=0
  Mux : Mux  Inputs=2
  Prod Scalare (P1-P0)*n : simulink/Math Operations/Dot Product  InputSameDT=on  OutDataType=sfix(16)  OutScaling=2^-10  DoSatur=off
  "Prod Scalare n*r " : simulink/Math Operations/Dot Product  InputSameDT=on  OutDataType=sfix(16)  OutScaling=2^-10  DoSatur=off
  Product : Product
  Sum : Sum  Inputs=|+-
  Sum1 : Sum  Inputs=|+-
  v_véhic (km/h){1..5} (5 alike) : Scope
  Pc : Outport
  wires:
  Gain/1 -> Mux/2
  Mux/1 -> Sum/2  "P0"
  Demux/1 -> Mux/1
  Demux/2 -> Gain/1
  P1/1 -> Demux/1, Sum/1, Sum1/1  "P1"
  r/1 -> "Prod Scalare n*r "/2, Product/1
  Prod Scalare (P1-P0)*n/1 -> v_véhic (km/h)3/1, Divide/1
  "Prod Scalare n*r "/1 -> v_véhic (km/h)1/1, Fcn/1
  Divide/1 -> v_véhic (km/h)4/1, Product/2
  Product/1 -> v_véhic (km/h)5/1, Sum1/2
  Sum1/1 -> Pc/1
  Sum/1 -> v_véhic (km/h)2/1, Prod Scalare (P1-P0)*n/1
  Fcn/1 -> Divide/2
  n/1 -> "Prod Scalare n*r "/1, Prod Scalare (P1-P0)*n/2

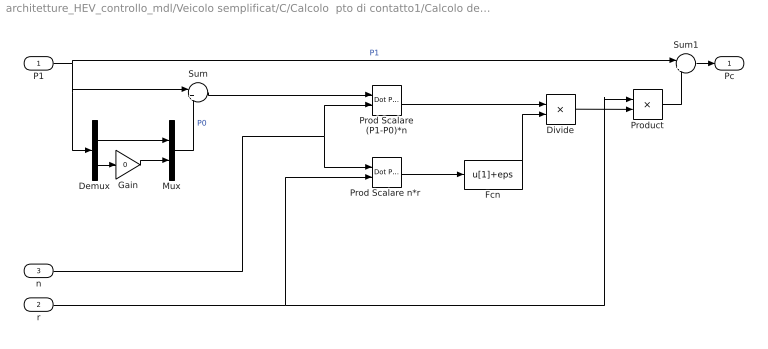
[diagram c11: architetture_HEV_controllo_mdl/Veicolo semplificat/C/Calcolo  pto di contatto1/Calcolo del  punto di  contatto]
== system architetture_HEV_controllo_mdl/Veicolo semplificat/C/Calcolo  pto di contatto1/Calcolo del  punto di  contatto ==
  P1 : Inport
  r : Inport  Port=2
  n : Inport  Port=3
  Demux : Demux  Outputs=2
  Divide : Product  Inputs=*/  OutScaling=2^-10
  Fcn : Fcn  Expr=u[1]+eps
  Gain : Gain  Gain=0
  Mux : Mux  Inputs=2
  Prod Scalare (P1-P0)*n : simulink/Math Operations/Dot Product  InputSameDT=on  OutDataType=sfix(16)  OutScaling=2^-10  DoSatur=off
  "Prod Scalare n*r " : simulink/Math Operations/Dot Product  InputSameDT=on  OutDataType=sfix(16)  OutScaling=2^-10  DoSatur=off
  Product : Product
  Sum : Sum  Inputs=|+-
  Sum1 : Sum  Inputs=|+-
  Pc : Outport
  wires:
  Gain/1 -> Mux/2
  Mux/1 -> Sum/2  "P0"
  Demux/1 -> Mux/1
  Demux/2 -> Gain/1
  P1/1 -> Demux/1, Sum/1, Sum1/1  "P1"
  r/1 -> "Prod Scalare n*r "/2, Product/1
  Prod Scalare (P1-P0)*n/1 -> Divide/1
  "Prod Scalare n*r "/1 -> Fcn/1
  Divide/1 -> Product/2
  Product/1 -> Sum1/2
  Sum1/1 -> Pc/1
  Sum/1 -> Prod Scalare (P1-P0)*n/1
  Fcn/1 -> Divide/2
  n/1 -> "Prod Scalare n*r "/1, Prod Scalare (P1-P0)*n/2

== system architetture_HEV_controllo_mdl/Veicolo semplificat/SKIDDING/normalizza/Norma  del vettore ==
  In1 : Inport
  Dot Product : simulink/Math Operations/Dot Product  InputSameDT=on  OutDataType=sfix(16)  OutScaling=2^-10  DoSatur=off
  Math Function : Math  Operator=sqrt
  Out1 : Outport
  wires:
  In1/1 -> Dot Product/1, Dot Product/2
  Dot Product/1 -> Math Function/1
  Math Function/1 -> Out1/1

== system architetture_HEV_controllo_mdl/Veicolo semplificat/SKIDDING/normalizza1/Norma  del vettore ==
  In1 : Inport
  Dot Product : simulink/Math Operations/Dot Product  InputSameDT=on  OutDataType=sfix(16)  OutScaling=2^-10  DoSatur=off
  Math Function : Math  Operator=sqrt
  Out1 : Outport
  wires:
  In1/1 -> Dot Product/1, Dot Product/2
  Dot Product/1 -> Math Function/1
  Math Function/1 -> Out1/1

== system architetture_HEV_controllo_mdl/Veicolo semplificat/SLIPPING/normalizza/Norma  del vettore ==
  In1 : Inport
  Dot Product : simulink/Math Operations/Dot Product  InputSameDT=on  OutDataType=sfix(16)  OutScaling=2^-10  DoSatur=off
  Math Function : Math  Operator=sqrt
  Out1 : Outport
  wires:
  In1/1 -> Dot Product/1, Dot Product/2
  Dot Product/1 -> Math Function/1
  Math Function/1 -> Out1/1

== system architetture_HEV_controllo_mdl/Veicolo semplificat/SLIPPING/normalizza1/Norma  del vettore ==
  In1 : Inport
  Dot Product : simulink/Math Operations/Dot Product  InputSameDT=on  OutDataType=sfix(16)  OutScaling=2^-10  DoSatur=off
  Math Function : Math  Operator=sqrt
  Out1 : Outport
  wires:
  In1/1 -> Dot Product/1, Dot Product/2
  Dot Product/1 -> Math Function/1
  Math Function/1 -> Out1/1
